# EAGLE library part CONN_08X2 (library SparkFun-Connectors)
Multi connection point. Often used as Generic Header-pin footprint for 0.1 inch spaced/style header connections You can populate with any combo of single row headers, but if you'd like an exact match, check this: Header - 2x8 (Male, 0.1") (PRT-13156) On any of the 0.1 inch spaced packages, you can populate with these: Break Away Headers - Straight (PRT-00116) Break Away Male Headers - Right Angle (PRT-00553) Female Headers (PRT-00115) Break Away Headers - Machine Pin (PRT-00117) Break Away Female Headers - Swiss Machine Pin (PRT-00743)
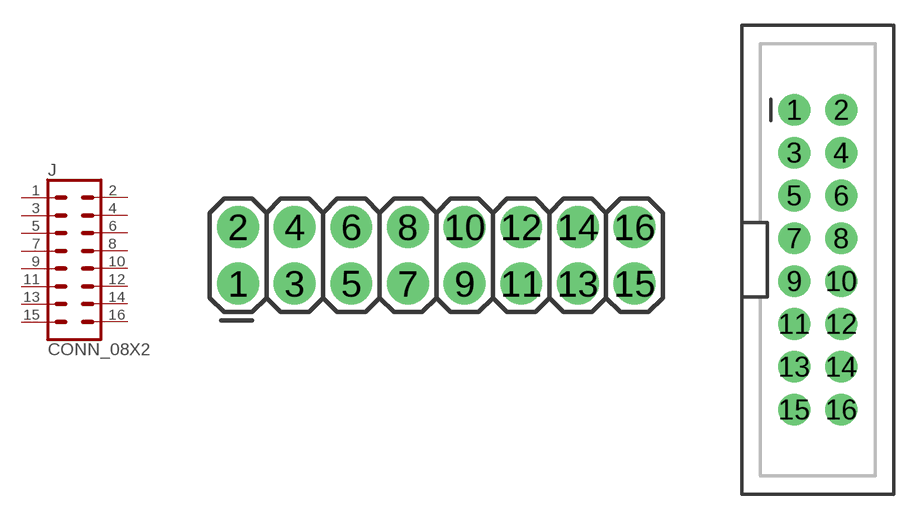
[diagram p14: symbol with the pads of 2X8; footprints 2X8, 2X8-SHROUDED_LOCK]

Designator prefix J

## CONN_08X2_HEADER  [2X8]
1  1  pas
2  2  pas
3  3  pas
4  4  pas
5  5  pas
6  6  pas
7  7  pas
8  8  pas
9  9  pas
10  10  pas
11  11  pas
12  12  pas
13  13  pas
14  14  pas
15  15  pas
16  16  pas

## CONN_08X2_SHROUD  [2X8-SHROUDED_LOCK]
Pads as for 2X8

## Footprint 2X8 (pad centres in mm)
Plated Through Hole - 2x8 Specifications: Pin count:16 Pin pitch:0.1" Example device(s): CONN_08x2
drill 1.016 pad 1.88: 1 0,0; 2 0,2.54; 3 2.54,0; 4 2.54,2.54; 5 5.08,0; 6 5.08,2.54; 7 7.62,0; 8 7.62,2.54; 9 10.16,0; 10 10.16,2.54; 11 12.7,0; 12 12.7,2.54; 13 15.24,0; 14 15.24,2.54; 15 17.78,0; 16 17.78,2.54

## Footprint 2X8-SHROUDED_LOCK (pad centres in mm)
drill 1.016 pad 1.88: 1 -1.397,8.89; 2 1.397,8.89; 3 -1.397,6.35; 4 1.397,6.35; 5 -1.397,3.81; 6 1.397,3.81; 7 -1.397,1.27; 8 1.397,1.27; 9 -1.397,-1.27; 10 1.397,-1.27; 11 -1.397,-3.81; 12 1.397,-3.81; 13 -1.397,-6.35; 14 1.397,-6.35; 15 -1.397,-8.89; 16 1.397,-8.89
